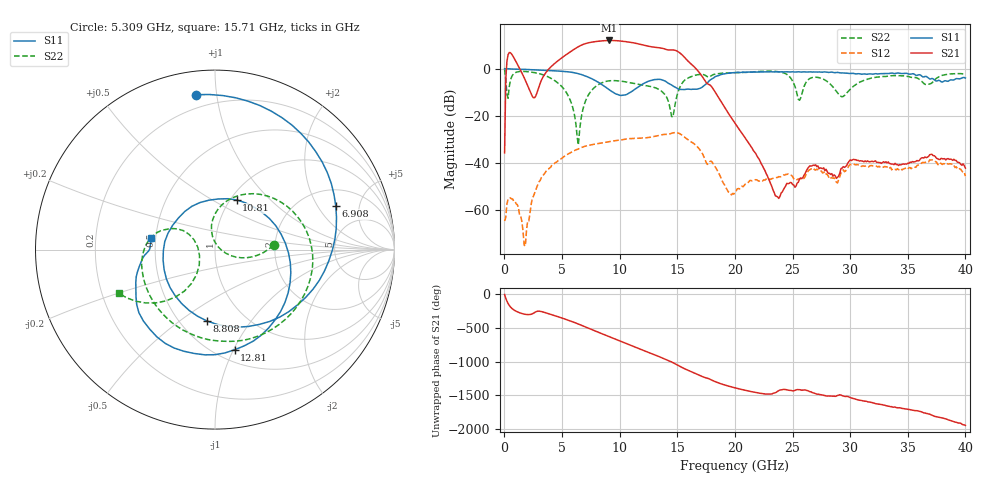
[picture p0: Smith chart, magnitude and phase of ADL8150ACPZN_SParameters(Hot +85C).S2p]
! Analog Devices, Inc.
! Device:	ADL8150ACPZN
! Description:	"GaAs, HBT, MMIC, Low Phase Noise Amplifier, 6 GHz to 14 GHz"
! Conditions:	Vcc = 5.0 V
!		Icc = 74 mA quiescent (Self-biased mode)
!		Pin = -20 dBm
!		Operating Temperature = +85 C (at package bottom)
! Product validation unit SN19 soldered down to Evaluation Board as shown on ADL8150-EVALZ User Guide. Board loss de-embedded from S21 magnitude.  All other RF measurements reference to RF coaxial connector.
! Frequency (GHz)	S11_Mag (dB)	S11_Phase (deg)	S21_Mag (dB)	S21_Phase (deg)	S12_Mag (dB)	S12_Phase (deg)	S22_Mag (dB)	S22_Phase (deg)
#  GHZ  S  DB  R 50
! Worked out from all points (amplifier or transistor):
!   401 points, 10 MHz to 40 GHz, reference 50 ohm
!   highest |S21| = 12.0 dB at 9.108 GHz (marker M1)
!   |S21| within 3 dB of that: 6.291 GHz to 13.23 GHz (6.936 GHz wide, 71.1 % of centre)
!   unconditionally stable (mu >= 1): start of sweep to end of sweep
!   at 6.608 GHz: K = 3.25, MAG = 13.8 dB, |S12| = -33.7 dB
!   at 20 GHz: K = 313.09, MAG = -13.4 dB, |S12| = -52.4 dB
!   at 40 GHz: K = 3108.05, MAG = -36.2 dB, |S12| = -45.8 dB
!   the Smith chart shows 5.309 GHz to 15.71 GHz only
!   S11 on the Smith chart (normalised r, x): 5.309 GHz: 0.12, +0.88; 6.908 GHz: 2.94, +2.93; 8.808 GHz: 0.67, -0.64; 10.81 GHz: 1.07, +0.65; 12.81 GHz: 0.61, -1.01; 15.71 GHz: 0.47, +0.07
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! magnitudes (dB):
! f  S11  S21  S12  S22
! 10 MHz  0.0  -35.8  -64.8  -0.2
! 409.9 MHz  -0.1  6.9  -55.5  -7.8
! 1.81 GHz  -0.3  -5.0  -75.5  -1.2
! 3.009 GHz  -0.6  -7.4  -48.1  -2.1
! 5.309 GHz  -1.2  5.8  -37.0  -9.7
! 6.308 GHz  -2.0  9.1  -34.4  -29.0
! 6.708 GHz  -2.6  10.1  -33.5  -19.5
! 6.908 GHz  -2.9  10.5  -33.1  -15.5
! 8.808 GHz  -8.0  12.0  -31.3  -5.4
! 9.108 GHz  -9.0  12.0  -31.0  -5.1
! 10.81 GHz  -10.4  11.3  -29.8  -5.9
! 12.81 GHz  -4.9  9.3  -29.0  -7.7
! 13.41 GHz  -4.5  8.9  -28.4  -8.9
! 14.61 GHz  -7.3  8.0  -27.3  -20.7
! 15.71 GHz  -8.8  4.4  -29.4  -4.6
! 20.1 GHz  -1.6  -24.0  -52.0  -1.7
! 23.7 GHz  -1.3  -54.5  -46.3  -1.2
! 25.6 GHz  -1.4  -47.0  -46.8  -13.4
! 26.7 GHz  -1.5  -41.3  -42.7  -3.8
! 29.3 GHz  -1.8  -42.3  -43.4  -12.0
! 33.4 GHz  -2.0  -40.3  -42.4  -3.1
! 40 GHz  -4.0  -42.3  -45.8  -2.3
